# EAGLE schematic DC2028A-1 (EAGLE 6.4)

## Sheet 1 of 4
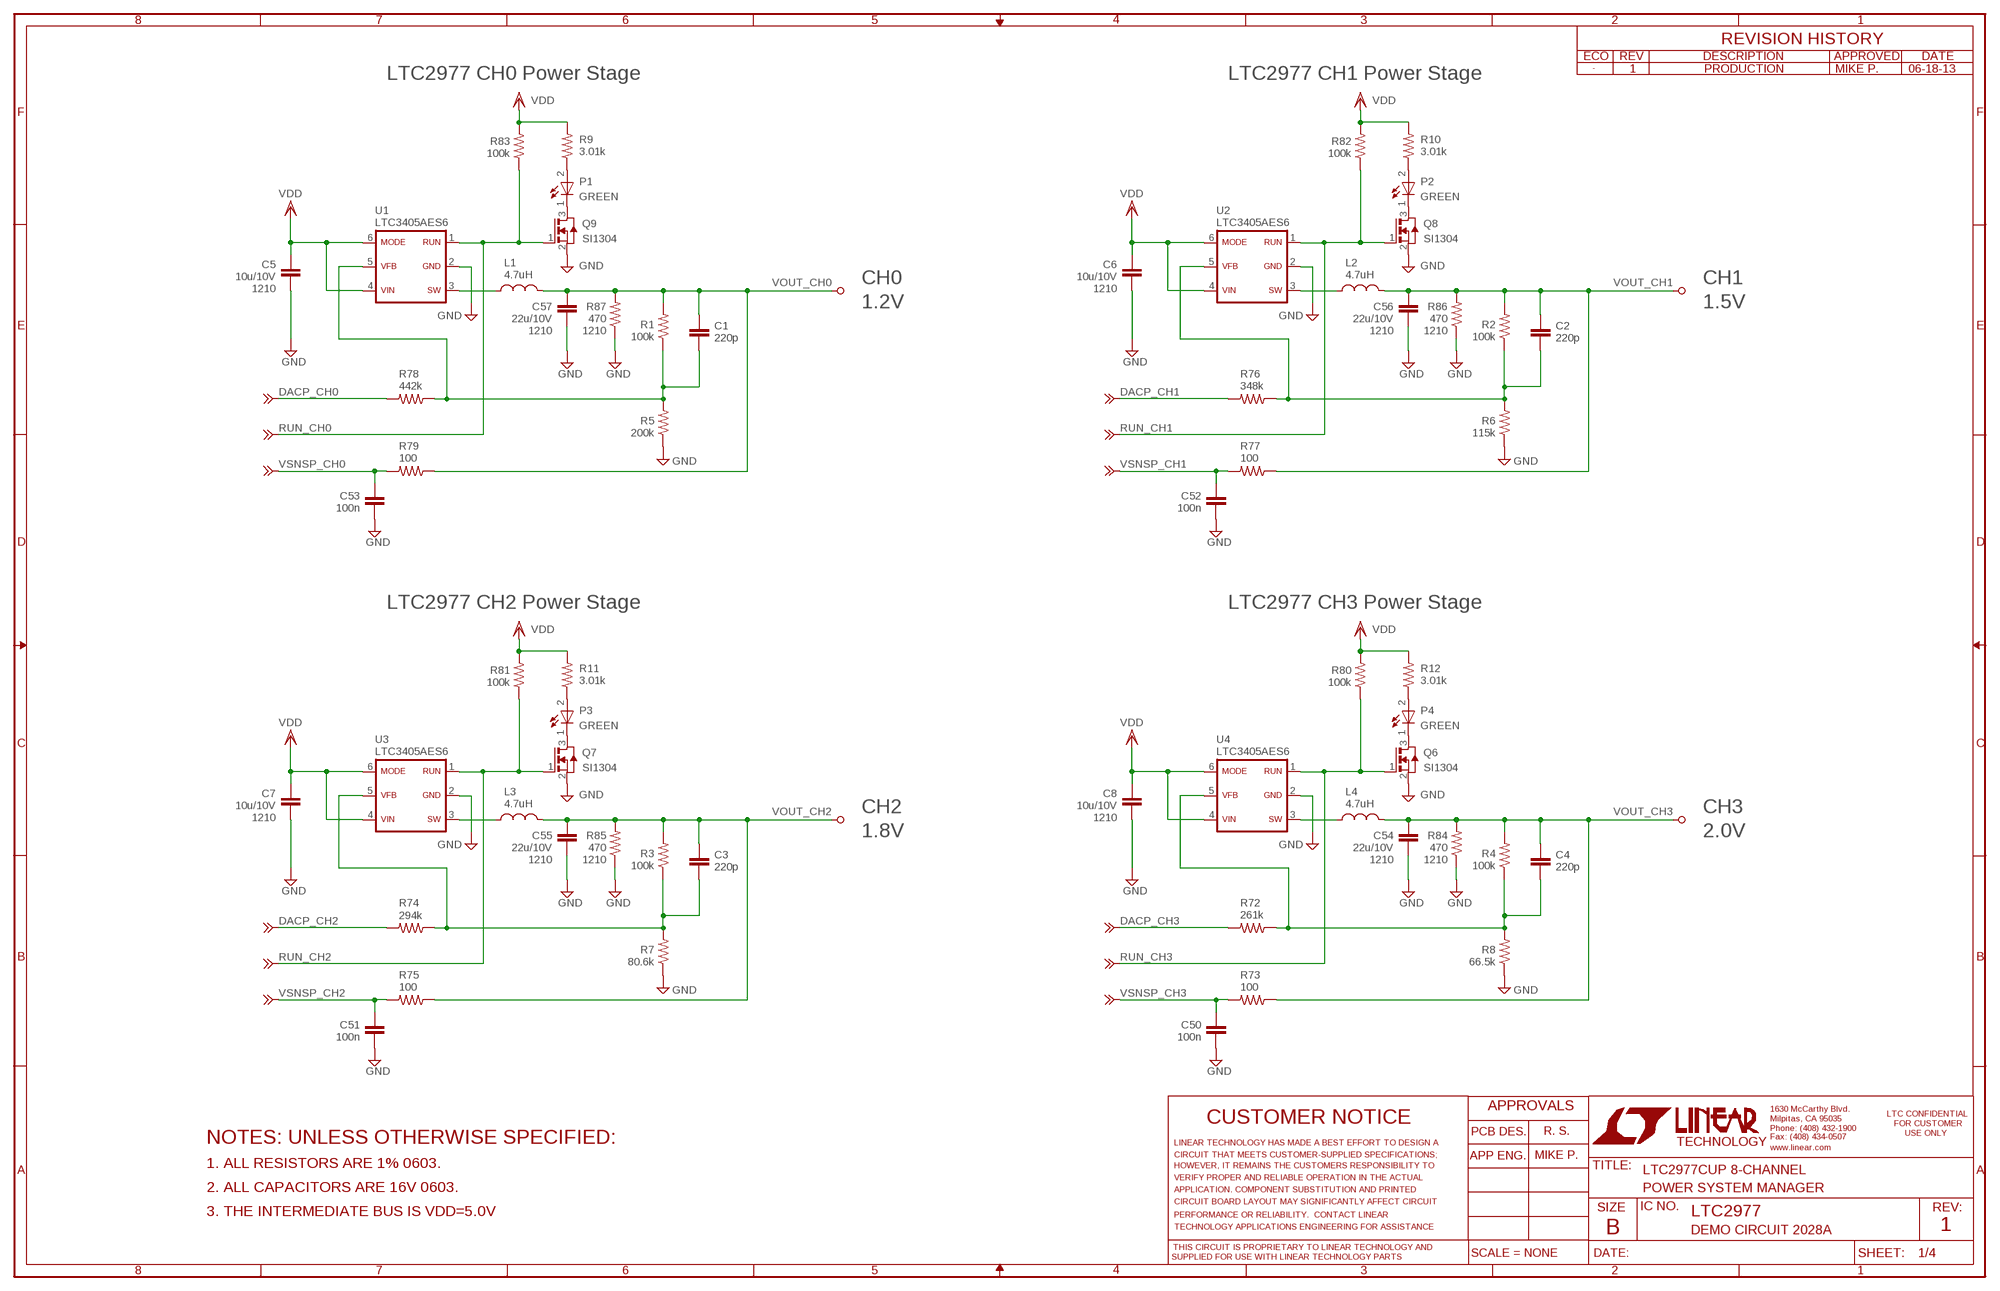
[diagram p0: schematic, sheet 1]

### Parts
C1  220p  CC0603_BOX  [C0603_BOX]
C2  220p  CC0603_BOX  [C0603_BOX]
C3  220p  CC0603_BOX  [C0603_BOX]
C4  220p  CC0603_BOX  [C0603_BOX]
C5  10u/10V  CC1210_BOX  [C1210_BOX]
C6  10u/10V  CC1210_BOX  [C1210_BOX]
C7  10u/10V  CC1210_BOX  [C1210_BOX]
C8  10u/10V  CC1210_BOX  [C1210_BOX]
C50  100n  CC0603_BOX  [C0603_BOX]
C51  100n  CC0603_BOX  [C0603_BOX]
C52  100n  CC0603_BOX  [C0603_BOX]
C53  100n  CC0603_BOX  [C0603_BOX]
C54  22u/10V  CC1210_BOX  [C1210_BOX]
C55  22u/10V  CC1210_BOX  [C1210_BOX]
C56  22u/10V  CC1210_BOX  [C1210_BOX]
C57  22u/10V  CC1210_BOX  [C1210_BOX]
L1  4.7uH  LL1210  [L1210]
L2  4.7uH  LL1210  [L1210]
L3  4.7uH  LL1210  [L1210]
L4  4.7uH  LL1210  [L1210]
P1  GREEN  LED-0603  [CHIPLED_0603]
P2  GREEN  LED-0603  [CHIPLED_0603]
P3  GREEN  LED-0603  [CHIPLED_0603]
P4  GREEN  LED-0603  [CHIPLED_0603]
Q6  SI1304  [SC70-3]
Q7  SI1304  [SC70-3]
Q8  SI1304  [SC70-3]
Q9  SI1304  [SC70-3]
R1  100k  RR0603_BOX  [R0603_BOX]
R2  100k  RR0603_BOX  [R0603_BOX]
R3  100k  RR0603_BOX  [R0603_BOX]
R4  100k  RR0603_BOX  [R0603_BOX]
R5  200k  RR0603_BOX  [R0603_BOX]
R6  115k  RR0603_BOX  [R0603_BOX]
R7  80.6k  RR0603_BOX  [R0603_BOX]
R8  66.5k  RR0603_BOX  [R0603_BOX]
R9  3.01k  RR0603_BOX  [R0603_BOX]
R10  3.01k  RR0603_BOX  [R0603_BOX]
R11  3.01k  RR0603_BOX  [R0603_BOX]
R12  3.01k  RR0603_BOX  [R0603_BOX]
R72  261k  RR0603_BOX  [R0603_BOX]
R73  100  RR0603_BOX  [R0603_BOX]
R74  294k  RR0603_BOX  [R0603_BOX]
R75  100  RR0603_BOX  [R0603_BOX]
R76  348k  RR0603_BOX  [R0603_BOX]
R77  100  RR0603_BOX  [R0603_BOX]
R78  442k  RR0603_BOX  [R0603_BOX]
R79  100  RR0603_BOX  [R0603_BOX]
R80  100k  RR0603_BOX  [R0603_BOX]
R81  100k  RR0603_BOX  [R0603_BOX]
R82  100k  RR0603_BOX  [R0603_BOX]
R83  100k  RR0603_BOX  [R0603_BOX]
R84  470  RR1210_BOX  [R1210_BOX]
R85  470  RR1210_BOX  [R1210_BOX]
R86  470  RR1210_BOX  [R1210_BOX]
R87  470  RR1210_BOX  [R1210_BOX]
TP3  TESTPOINT_BIG  [TP1]
TP4  TESTPOINT_BIG  [TP1]
TP5  TESTPOINT_BIG  [TP1]
TP6  TESTPOINT_BIG  [TP1]
U1  LTC3405AES6  LTC3405ES6  [SOT-23-6]
U2  LTC3405AES6  LTC3405ES6  [SOT-23-6]
U3  LTC3405AES6  LTC3405ES6  [SOT-23-6]
U4  LTC3405AES6  LTC3405ES6  [SOT-23-6]
VSNSN1  TESPOINT_SMD  TESPOINT_SMDVIA  [VIA]
VSNSN2  TESPOINT_SMD  TESPOINT_SMDVIA  [VIA]
VSNSN3  TESPOINT_SMD  TESPOINT_SMDVIA  [VIA]
VSNSN4  TESPOINT_SMD  TESPOINT_SMDVIA  [VIA]
VSNSN17  TESPOINT_SMD  TESPOINT_SMDVIA  [VIA]
VSNSN18  TESPOINT_SMD  TESPOINT_SMDVIA  [VIA]
VSNSN19  TESPOINT_SMD  TESPOINT_SMDVIA  [VIA]
VSNSN20  TESPOINT_SMD  TESPOINT_SMDVIA  [VIA]
VSNSN21  TESPOINT_SMD  TESPOINT_SMDVIA  [VIA]
VSNSN22  TESPOINT_SMD  TESPOINT_SMDVIA  [VIA]
VSNSN23  TESPOINT_SMD  TESPOINT_SMDVIA  [VIA]
VSNSN24  TESPOINT_SMD  TESPOINT_SMDVIA  [VIA]

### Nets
DACP_CH0: R78.2 VSNSN23.1 ; also sheet 3
DACP_CH1: R76.2 VSNSN21.1 ; also sheet 3
DACP_CH2: R74.2 VSNSN19.1 ; also sheet 3
DACP_CH3: R72.2 VSNSN17.1 ; also sheet 3
GND: C5.2 C6.2 C7.2 C8.2 C50.1 C51.1 C52.1 C53.1 C54.2 C55.2 C56.2 C57.2 Q6.2(S) Q7.2(S) Q8.2(S) Q9.2(S) R5.1 R6.1 R7.1 R8.1 R84.1 R85.1 R86.1 R87.1 U1.2 U2.2 U3.2 U4.2 ; also sheet 2,3,4
N$6: P1.P(A) R9.1
N$7: P1.N(C) Q9.3(D)
N$8: P2.P(A) R10.1
N$9: P2.N(C) Q8.3(D)
N$10: P3.P(A) R11.1
N$11: P3.N(C) Q7.3(D)
N$12: P4.P(A) R12.1
N$13: P4.N(C) Q6.3(D)
RUN_CH0: Q9.1(G) R83.1 U1.1 VSNSN1.1 ; also sheet 3
RUN_CH1: Q8.1(G) R82.1 U2.1 VSNSN2.1 ; also sheet 3
RUN_CH2: Q7.1(G) R81.1 U3.1 VSNSN3.1 ; also sheet 3
RUN_CH3: Q6.1(G) R80.1 U4.1 VSNSN4.1 ; also sheet 3
SW1: L1.1 U1.3
SW2: L2.1 U2.3
SW3: L3.1 U3.3
SW4: L4.1 U4.3
VDD: C5.1 C6.1 C7.1 C8.1 R9.2 R10.2 R11.2 R12.2 R80.2 R81.2 R82.2 R83.2 U1.4 U1.6 U2.4 U2.6 U3.4 U3.6 U4.4 U4.6 ; also sheet 2,3,4
VFB1: C1.2 R1.1 R5.2 R78.1 U1.5
VFB2: C2.2 R2.1 R6.2 R76.1 U2.5
VFB3: C3.2 R3.1 R7.2 R74.1 U3.5
VFB12: C4.2 R4.1 R8.2 R72.1 U4.5
VOUT_CH0: C1.1 C57.1 L1.2 R1.2 R79.1 R87.2 TP3.TP
VOUT_CH1: C2.1 C56.1 L2.2 R2.2 R77.1 R86.2 TP4.TP
VOUT_CH2: C3.1 C55.1 L3.2 R3.2 R75.1 R85.2 TP5.TP
VOUT_CH3: C4.1 C54.1 L4.2 R4.2 R73.1 R84.2 TP6.TP
VSNSP_CH0: C53.2 R79.2 VSNSN24.1 ; also sheet 3
VSNSP_CH1: C52.2 R77.2 VSNSN22.1 ; also sheet 3
VSNSP_CH2: C51.2 R75.2 VSNSN20.1 ; also sheet 3
VSNSP_CH3: C50.2 R73.2 VSNSN18.1 ; also sheet 3

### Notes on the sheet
- 1 | PRODUCTION | MIKE P. | 06-18-13
- LTC2977 CH0 Power Stage | LTC2977 CH1 Power Stage
- 1210 | CH0 | 1210 | CH1
- 1.2V | 1.5V
- 1210 | 1210 | 1210 | 1210
- LTC2977 CH2 Power Stage | LTC2977 CH3 Power Stage
- 1210 | CH2 | 1210 | CH3
- 1.8V | 2.0V
- 1210 | 1210 | 1210 | 1210
- R. S.
- NOTES: UNLESS OTHERWISE SPECIFIED:
- MIKE P.
- 1. ALL RESISTORS ARE 1% 0603.
- LTC2977CUP 8-CHANNEL
- 2. ALL CAPACITORS ARE 16V 0603. | POWER SYSTEM MANAGER
- 3. THE INTERMEDIATE BUS IS VDD=5.0V | LTC2977
- DEMO CIRCUIT 2028A | 1

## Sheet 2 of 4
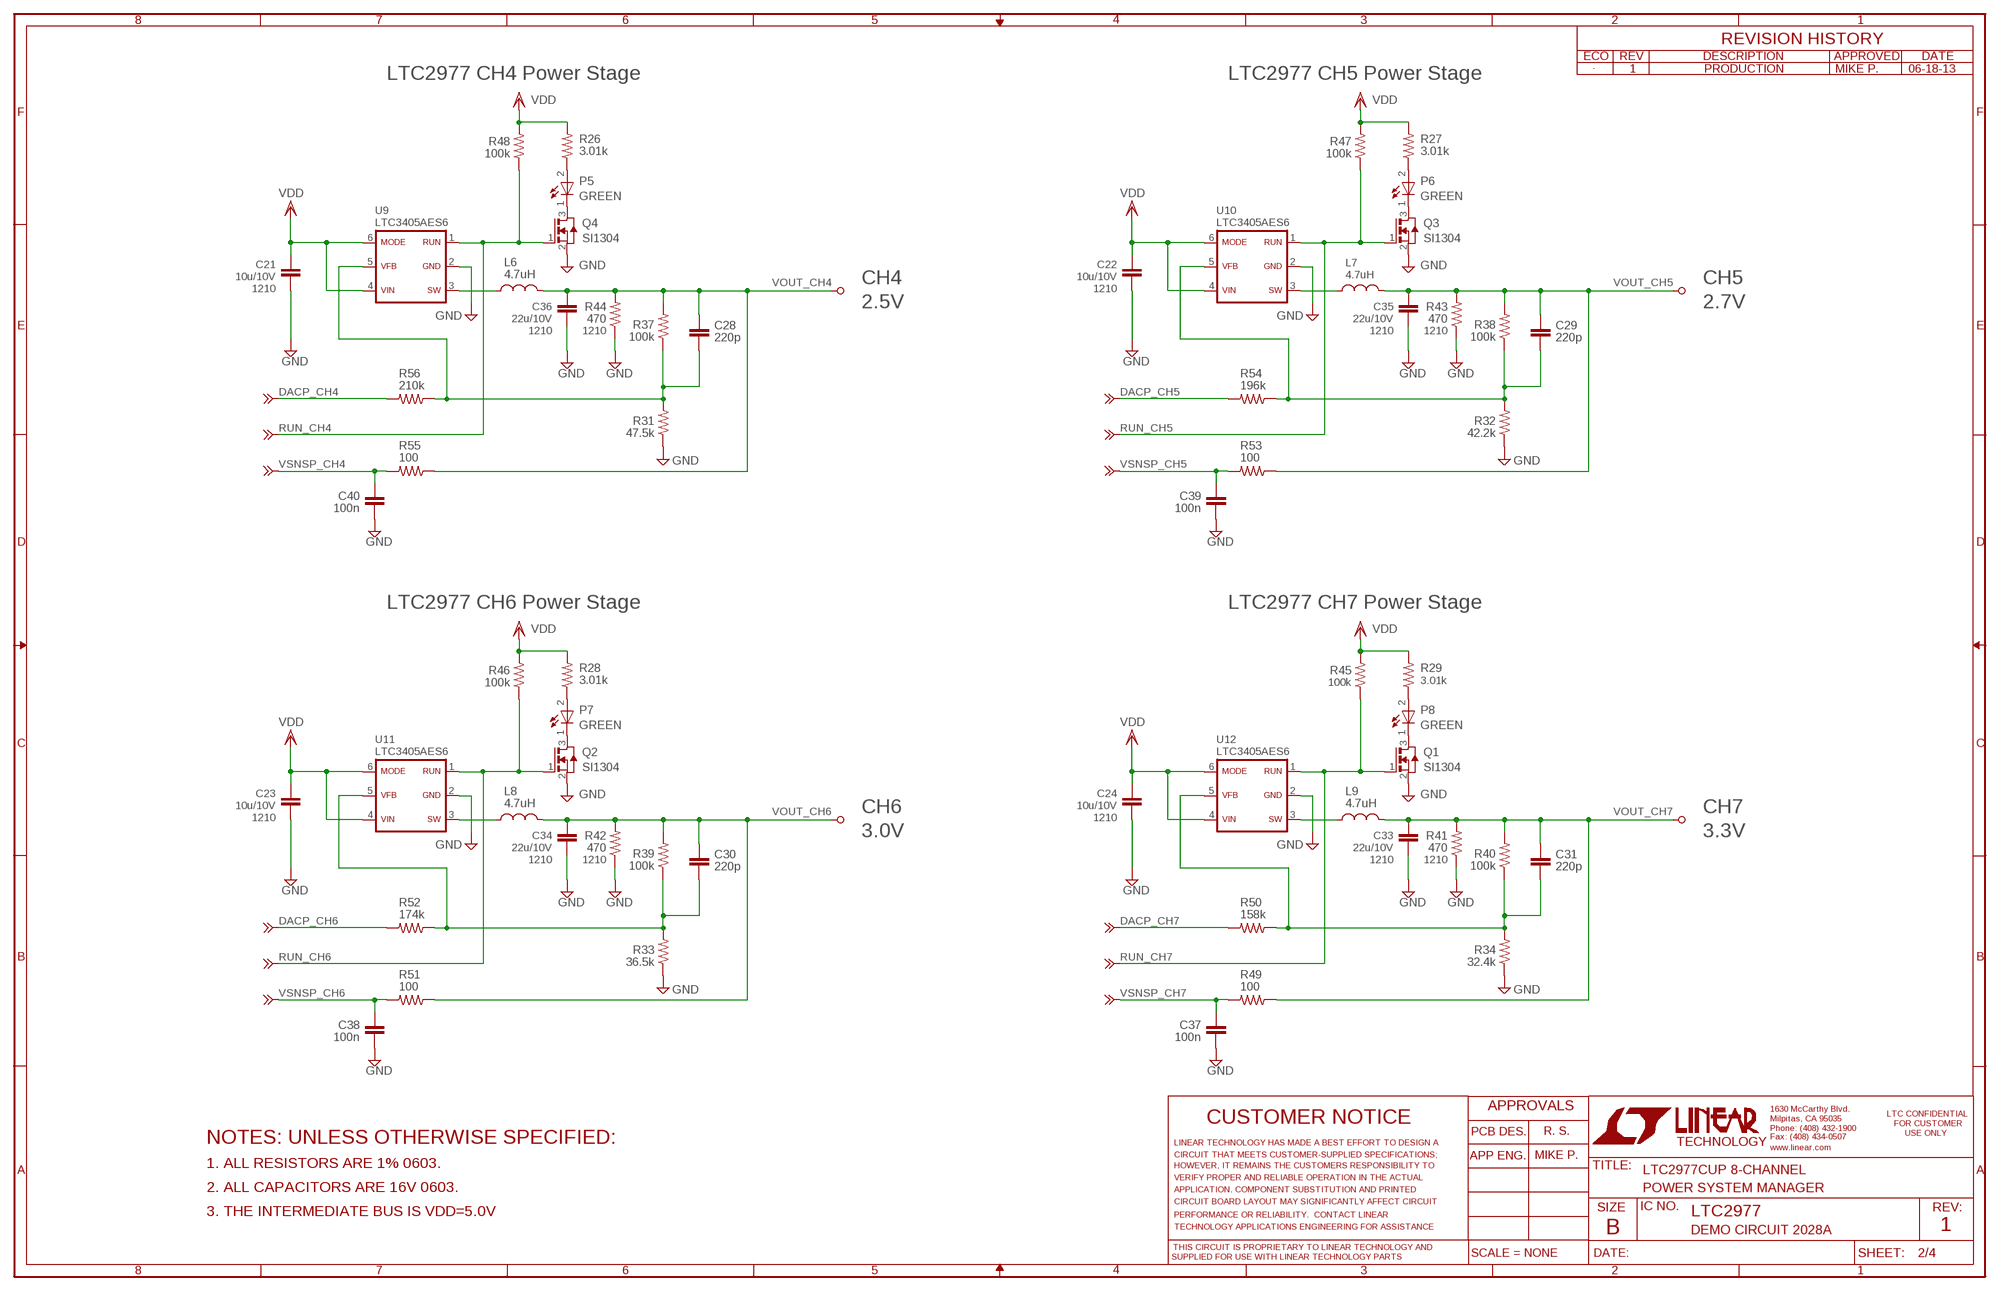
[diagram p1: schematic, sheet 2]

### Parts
C21  10u/10V  CC1210_BOX  [C1210_BOX]
C22  10u/10V  CC1210_BOX  [C1210_BOX]
C23  10u/10V  CC1210_BOX  [C1210_BOX]
C24  10u/10V  CC1210_BOX  [C1210_BOX]
C28  220p  CC0603_BOX  [C0603_BOX]
C29  220p  CC0603_BOX  [C0603_BOX]
C30  220p  CC0603_BOX  [C0603_BOX]
C31  220p  CC0603_BOX  [C0603_BOX]
C33  22u/10V  CC1210_BOX  [C1210_BOX]
C34  22u/10V  CC1210_BOX  [C1210_BOX]
C35  22u/10V  CC1210_BOX  [C1210_BOX]
C36  22u/10V  CC1210_BOX  [C1210_BOX]
C37  100n  CC0603_BOX  [C0603_BOX]
C38  100n  CC0603_BOX  [C0603_BOX]
C39  100n  CC0603_BOX  [C0603_BOX]
C40  100n  CC0603_BOX  [C0603_BOX]
L6  4.7uH  LL1210  [L1210]
L7  4.7uH  LL1210  [L1210]
L8  4.7uH  LL1210  [L1210]
L9  4.7uH  LL1210  [L1210]
P5  GREEN  LED-0603  [CHIPLED_0603]
P6  GREEN  LED-0603  [CHIPLED_0603]
P7  GREEN  LED-0603  [CHIPLED_0603]
P8  GREEN  LED-0603  [CHIPLED_0603]
Q1  SI1304  [SC70-3]
Q2  SI1304  [SC70-3]
Q3  SI1304  [SC70-3]
Q4  SI1304  [SC70-3]
R26  3.01k  RR0603_BOX  [R0603_BOX]
R27  3.01k  RR0603_BOX  [R0603_BOX]
R28  3.01k  RR0603_BOX  [R0603_BOX]
R29  3.01k  RR0603_BOX  [R0603_BOX]
R31  47.5k  RR0603_BOX  [R0603_BOX]
R32  42.2k  RR0603_BOX  [R0603_BOX]
R33  36.5k  RR0603_BOX  [R0603_BOX]
R34  32.4k  RR0603_BOX  [R0603_BOX]
R37  100k  RR0603_BOX  [R0603_BOX]
R38  100k  RR0603_BOX  [R0603_BOX]
R39  100k  RR0603_BOX  [R0603_BOX]
R40  100k  RR0603_BOX  [R0603_BOX]
R41  470  RR1210_BOX  [R1210_BOX]
R42  470  RR1210_BOX  [R1210_BOX]
R43  470  RR1210_BOX  [R1210_BOX]
R44  470  RR1210_BOX  [R1210_BOX]
R45  100k  RR0603_BOX  [R0603_BOX]
R46  100k  RR0603_BOX  [R0603_BOX]
R47  100k  RR0603_BOX  [R0603_BOX]
R48  100k  RR0603_BOX  [R0603_BOX]
R49  100  RR0603_BOX  [R0603_BOX]
R50  158k  RR0603_BOX  [R0603_BOX]
R51  100  RR0603_BOX  [R0603_BOX]
R52  174k  RR0603_BOX  [R0603_BOX]
R53  100  RR0603_BOX  [R0603_BOX]
R54  196k  RR0603_BOX  [R0603_BOX]
R55  100  RR0603_BOX  [R0603_BOX]
R56  210k  RR0603_BOX  [R0603_BOX]
TP17  TESTPOINT_BIG  [TP1]
TP18  TESTPOINT_BIG  [TP1]
TP19  TESTPOINT_BIG  [TP1]
TP20  TESTPOINT_BIG  [TP1]
U9  LTC3405AES6  LTC3405ES6  [SOT-23-6]
U10  LTC3405AES6  LTC3405ES6  [SOT-23-6]
U11  LTC3405AES6  LTC3405ES6  [SOT-23-6]
U12  LTC3405AES6  LTC3405ES6  [SOT-23-6]
VSNSN5  TESPOINT_SMD  TESPOINT_SMDVIA  [VIA]
VSNSN6  TESPOINT_SMD  TESPOINT_SMDVIA  [VIA]
VSNSN7  TESPOINT_SMD  TESPOINT_SMDVIA  [VIA]
VSNSN8  TESPOINT_SMD  TESPOINT_SMDVIA  [VIA]
VSNSN9  TESPOINT_SMD  TESPOINT_SMDVIA  [VIA]
VSNSN10  TESPOINT_SMD  TESPOINT_SMDVIA  [VIA]
VSNSN11  TESPOINT_SMD  TESPOINT_SMDVIA  [VIA]
VSNSN12  TESPOINT_SMD  TESPOINT_SMDVIA  [VIA]
VSNSN13  TESPOINT_SMD  TESPOINT_SMDVIA  [VIA]
VSNSN14  TESPOINT_SMD  TESPOINT_SMDVIA  [VIA]
VSNSN15  TESPOINT_SMD  TESPOINT_SMDVIA  [VIA]
VSNSN16  TESPOINT_SMD  TESPOINT_SMDVIA  [VIA]

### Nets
DACP_CH4: R56.2 VSNSN16.1 ; also sheet 3
DACP_CH5: R54.2 VSNSN14.1 ; also sheet 3
DACP_CH6: R52.2 VSNSN12.1 ; also sheet 3
DACP_CH7: R50.2 VSNSN10.1 ; also sheet 3
GND: C21.2 C22.2 C23.2 C24.2 C33.2 C34.2 C35.2 C36.2 C37.1 C38.1 C39.1 C40.1 Q1.2(S) Q2.2(S) Q3.2(S) Q4.2(S) R31.1 R32.1 R33.1 R34.1 R41.1 R42.1 R43.1 R44.1 U9.2 U10.2 U11.2 U12.2 ; also sheet 1,3,4
N$29: P5.P(A) R26.1
N$30: P5.N(C) Q4.3(D)
N$31: P6.P(A) R27.1
N$32: P6.N(C) Q3.3(D)
N$33: P7.P(A) R28.1
N$34: P7.N(C) Q2.3(D)
N$35: P8.P(A) R29.1
N$36: P8.N(C) Q1.3(D)
RUN_CH4: Q4.1(G) R48.1 U9.1 VSNSN5.1 ; also sheet 3
RUN_CH5: Q3.1(G) R47.1 U10.1 VSNSN6.1 ; also sheet 3
RUN_CH6: Q2.1(G) R46.1 U11.1 VSNSN7.1 ; also sheet 3
RUN_CH7: Q1.1(G) R45.1 U12.1 VSNSN8.1 ; also sheet 3
SW11: L6.1 U9.3
SW12: L7.1 U10.3
SW13: L8.1 U11.3
SW14: L9.1 U12.3
VDD: C21.1 C22.1 C23.1 C24.1 R26.2 R27.2 R28.2 R29.2 R45.2 R46.2 R47.2 R48.2 U9.4 U9.6 U10.4 U10.6 U11.4 U11.6 U12.4 U12.6 ; also sheet 1,3,4
VFB4: C28.2 R31.2 R37.1 R56.1 U9.5
VFB5: C29.2 R32.2 R38.1 R54.1 U10.5
VFB6: C30.2 R33.2 R39.1 R52.1 U11.5
VFB7: C31.2 R34.2 R40.1 R50.1 U12.5
VOUT_CH4: C28.1 C36.1 L6.2 R37.2 R44.2 R55.1 TP17.TP
VOUT_CH5: C29.1 C35.1 L7.2 R38.2 R43.2 R53.1 TP18.TP
VOUT_CH6: C30.1 C34.1 L8.2 R39.2 R42.2 R51.1 TP19.TP
VOUT_CH7: C31.1 C33.1 L9.2 R40.2 R41.2 R49.1 TP20.TP ; also sheet 3
VSNSP_CH4: C40.2 R55.2 VSNSN15.1 ; also sheet 3
VSNSP_CH5: C39.2 R53.2 VSNSN13.1 ; also sheet 3
VSNSP_CH6: C38.2 R51.2 VSNSN11.1 ; also sheet 3
VSNSP_CH7: C37.2 R49.2 VSNSN9.1 ; also sheet 3

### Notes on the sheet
- 1 | PRODUCTION | MIKE P. | 06-18-13
- LTC2977 CH4 Power Stage | LTC2977 CH5 Power Stage
- 1210 | CH4 | 1210 | CH5
- 2.5V | 2.7V
- 1210 | 1210 | 1210 | 1210
- LTC2977 CH6 Power Stage | LTC2977 CH7 Power Stage
- 1210 | CH6 | 1210 | CH7
- 3.0V | 3.3V
- 1210 | 1210 | 1210 | 1210
- R. S.
- NOTES: UNLESS OTHERWISE SPECIFIED:
- MIKE P.
- 1. ALL RESISTORS ARE 1% 0603.
- LTC2977CUP 8-CHANNEL
- 2. ALL CAPACITORS ARE 16V 0603. | POWER SYSTEM MANAGER
- 3. THE INTERMEDIATE BUS IS VDD=5.0V | LTC2977
- DEMO CIRCUIT 2028A | 1

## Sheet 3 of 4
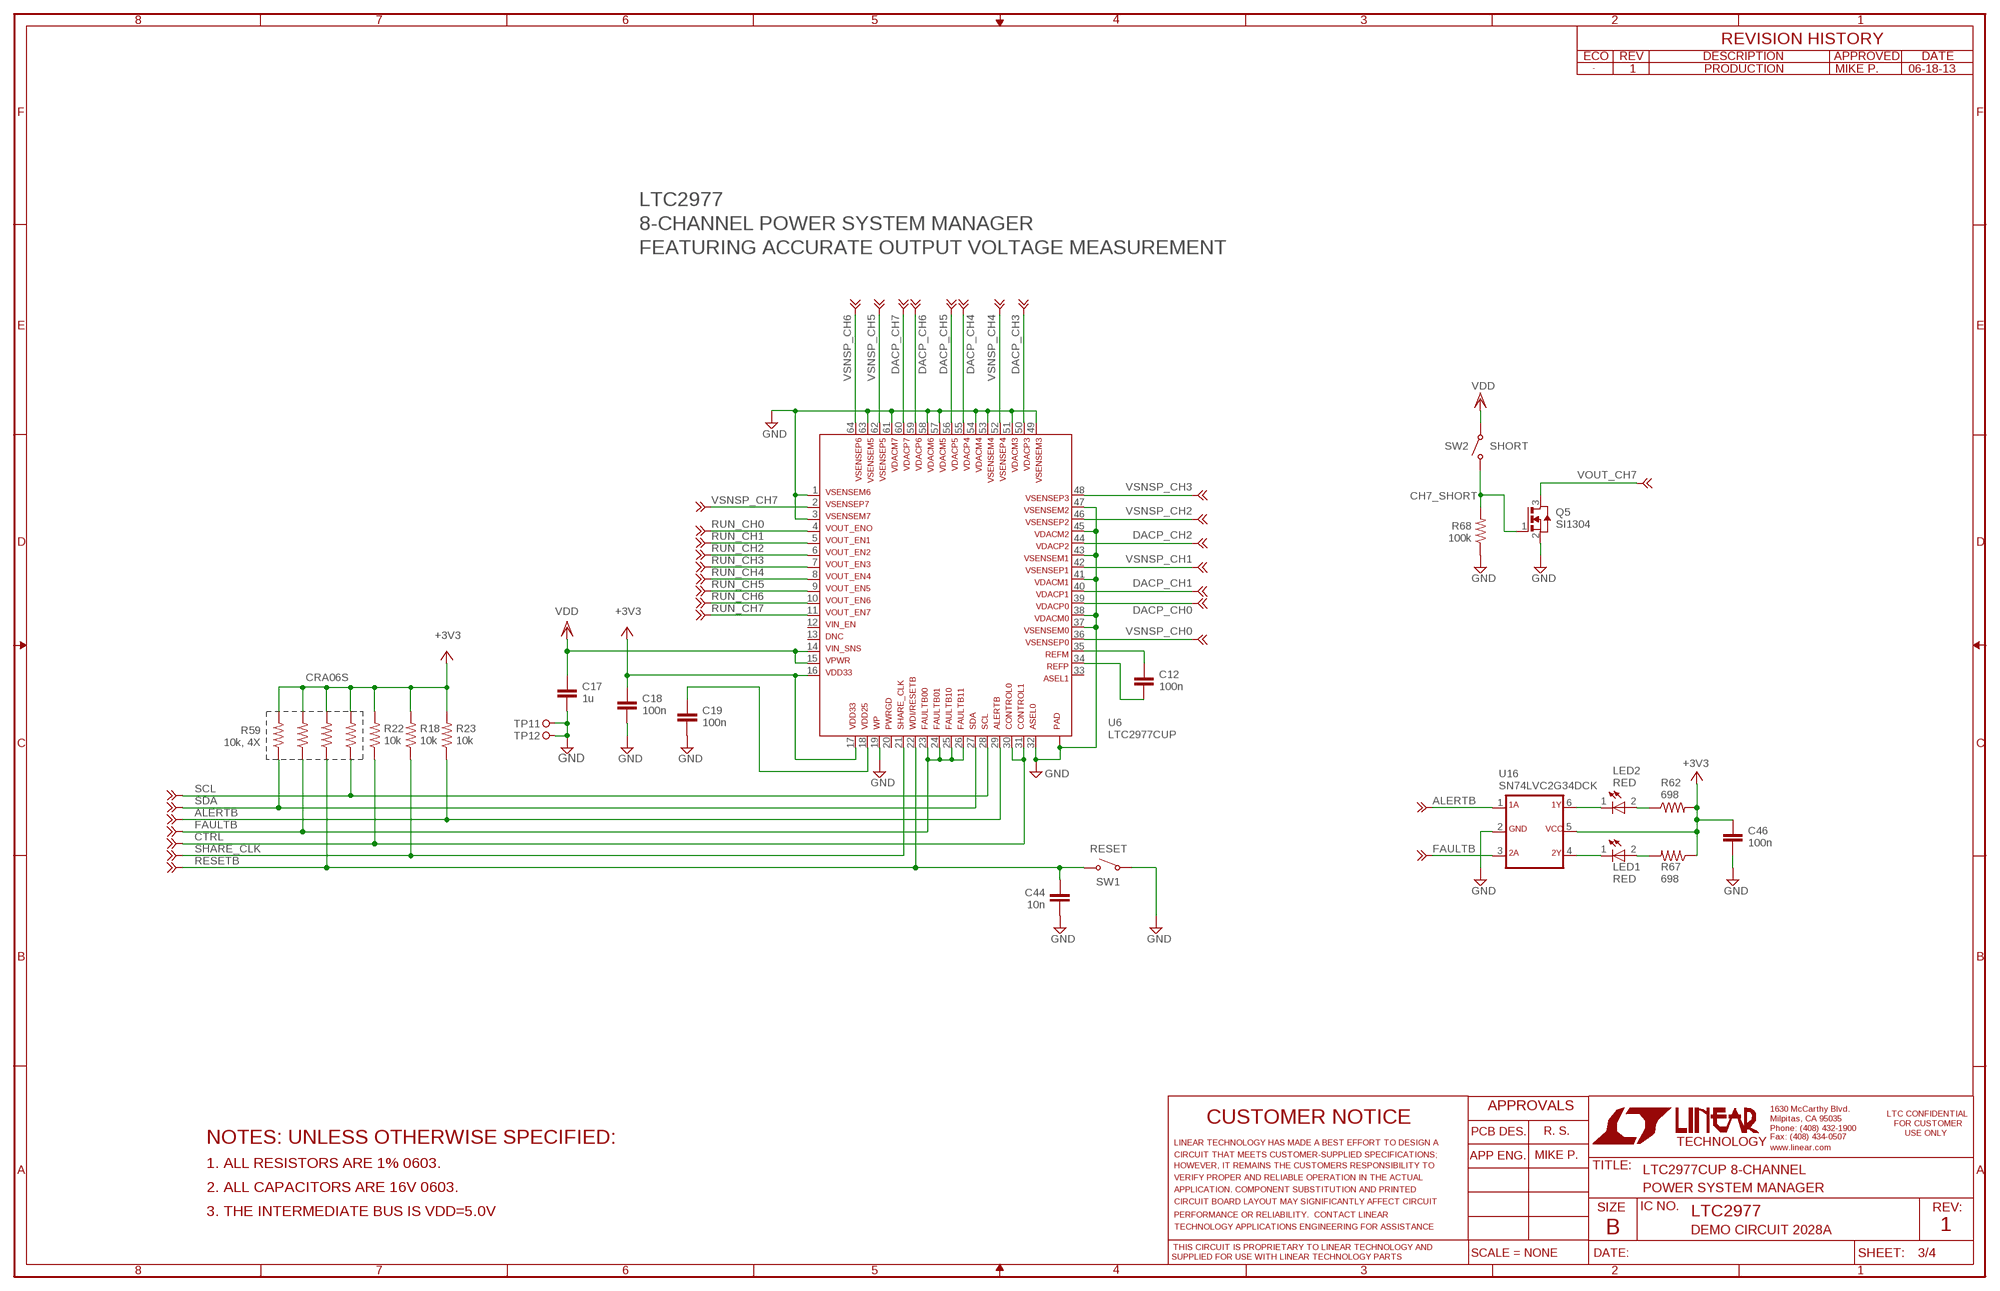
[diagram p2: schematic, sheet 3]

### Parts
C12  100n  CC0603_BOX  [C0603_BOX]
C17  1u  CC0603_BOX  [C0603_BOX]
C18  100n  CC0603_BOX  [C0603_BOX]
C19  100n  CC0603_BOX  [C0603_BOX]
C44  10n  CC0603_BOX  [C0603_BOX]
C46  100n  CC0603_BOX  [C0603_BOX]
LED1  RED  LED-0603  [CHIPLED_0603]
LED2  RED  LED-0603  [CHIPLED_0603]
Q5  SI1304  [SC70-3]
R18  10k  RR0603_BOX  [R0603_BOX]
R22  10k  RR0603_BOX  [R0603_BOX]
R23  10k  RR0603_BOX  [R0603_BOX]
R59  10k, 4X  R_ARRAY_4X_CRA06S  [R_VISHAY_CRA06S]
R62  698  RR0603_BOX  [R0603_BOX]
R67  698  RR0603_BOX  [R0603_BOX]
R68  100k  RR0603_BOX  [R0603_BOX]
SW1  PTS635SL25SMTR LFS  SWITCH_PTS635  [SWITCH_PTS635]
SW2  PTS635SK25SMTR LFS  SWITCH_PTS635  [SWITCH_PTS635]
TP11  TESTPOINT_BIG  [TP1]
TP12  TESTPOINT_BIG  [TP1]
U6  LTC2977CUP  LTC2978CUP  [QFN64_9X9]
U16  SN74LVC2G34DCK  [SC70-6]

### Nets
+3V3: C18.2 C46.1 R18.2 R22.2 R23.2 R59.R1_2 R59.R2_2 R59.R3_2 R59.R4_2 R62.2 R67.1 U6.16 U6.17 U16.5 ; also sheet 4
ALERTB: R23.1 U6.29 U16.1 ; also sheet 4
CH7_SHORT: Q5.1(G) R68.2 SW2.SW1 ; also sheet 4
CTRL: R22.1 U6.30 U6.31 ; also sheet 4
DACP_CH0: U6.39 ; also sheet 1
DACP_CH1: U6.40 ; also sheet 1
DACP_CH2: U6.44 ; also sheet 1
DACP_CH3: U6.50 ; also sheet 1
DACP_CH4: U6.55 ; also sheet 2
DACP_CH5: U6.56 ; also sheet 2
DACP_CH6: U6.59 ; also sheet 2
DACP_CH7: U6.60 ; also sheet 2
FAULTB: R59.R2_1 U6.23 U6.24 U6.25 U6.26 U16.3 ; also sheet 4
GND: C17.1 C18.1 C19.1 C44.2 C46.2 Q5.2(S) R68.1 SW1.SW2 TP11.TP TP12.TP U6.1 U6.3 U6.19 U6.32 U6.37 U6.38 U6.41 U6.43 U6.45 U6.47 U6.49 U6.51 U6.53 U6.54 U6.57 U6.58 U6.61 U6.63 U6.PAD1 U6.PAD2 U6.PAD3 U6.PAD4 U16.2 ; also sheet 1,2,4
N$3: LED1.P(A) R67.2
N$53: C12.1 U6.35
N$54: C12.2 U6.34
N$56: C19.2 U6.18
N$57: LED2.P(A) R62.1
N$58: LED1.N(C) U16.4
N$60: LED2.N(C) U16.6
RESETB: C44.1 R59.R3_1 SW1.SW1 U6.22 ; also sheet 4
RUN_CH0: U6.4 ; also sheet 1
RUN_CH1: U6.5 ; also sheet 1
RUN_CH2: U6.6 ; also sheet 1
RUN_CH3: U6.7 ; also sheet 1
RUN_CH4: U6.8 ; also sheet 2
RUN_CH5: U6.9 ; also sheet 2
RUN_CH6: U6.10 ; also sheet 2
RUN_CH7: U6.11 ; also sheet 2
SCL: R59.R4_1 U6.28 ; also sheet 4
SDA: R59.R1_1 U6.27 ; also sheet 4
SHARE_CLK: R18.1 U6.21 ; also sheet 4
VDD: C17.2 SW2.SW2 U6.14 U6.15 ; also sheet 1,2,4
VOUT_CH7: Q5.3(D) ; also sheet 2
VSNSP_CH0: U6.36 ; also sheet 1
VSNSP_CH1: U6.42 ; also sheet 1
VSNSP_CH2: U6.46 ; also sheet 1
VSNSP_CH3: U6.48 ; also sheet 1
VSNSP_CH4: U6.52 ; also sheet 2
VSNSP_CH5: U6.62 ; also sheet 2
VSNSP_CH6: U6.64 ; also sheet 2
VSNSP_CH7: U6.2 ; also sheet 2
Unconnected: U6.12 U6.13 U6.20 U6.33

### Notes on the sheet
- 1 | PRODUCTION | MIKE P. | 06-18-13
- LTC2977
- 8-CHANNEL POWER SYSTEM MANAGER
- FEATURING ACCURATE OUTPUT VOLTAGE MEASUREMENT
- SHORT
- CRA06S
- RESET
- R. S.
- NOTES: UNLESS OTHERWISE SPECIFIED:
- MIKE P.
- 1. ALL RESISTORS ARE 1% 0603.
- LTC2977CUP 8-CHANNEL
- 2. ALL CAPACITORS ARE 16V 0603. | POWER SYSTEM MANAGER
- 3. THE INTERMEDIATE BUS IS VDD=5.0V | LTC2977
- DEMO CIRCUIT 2028A | 1

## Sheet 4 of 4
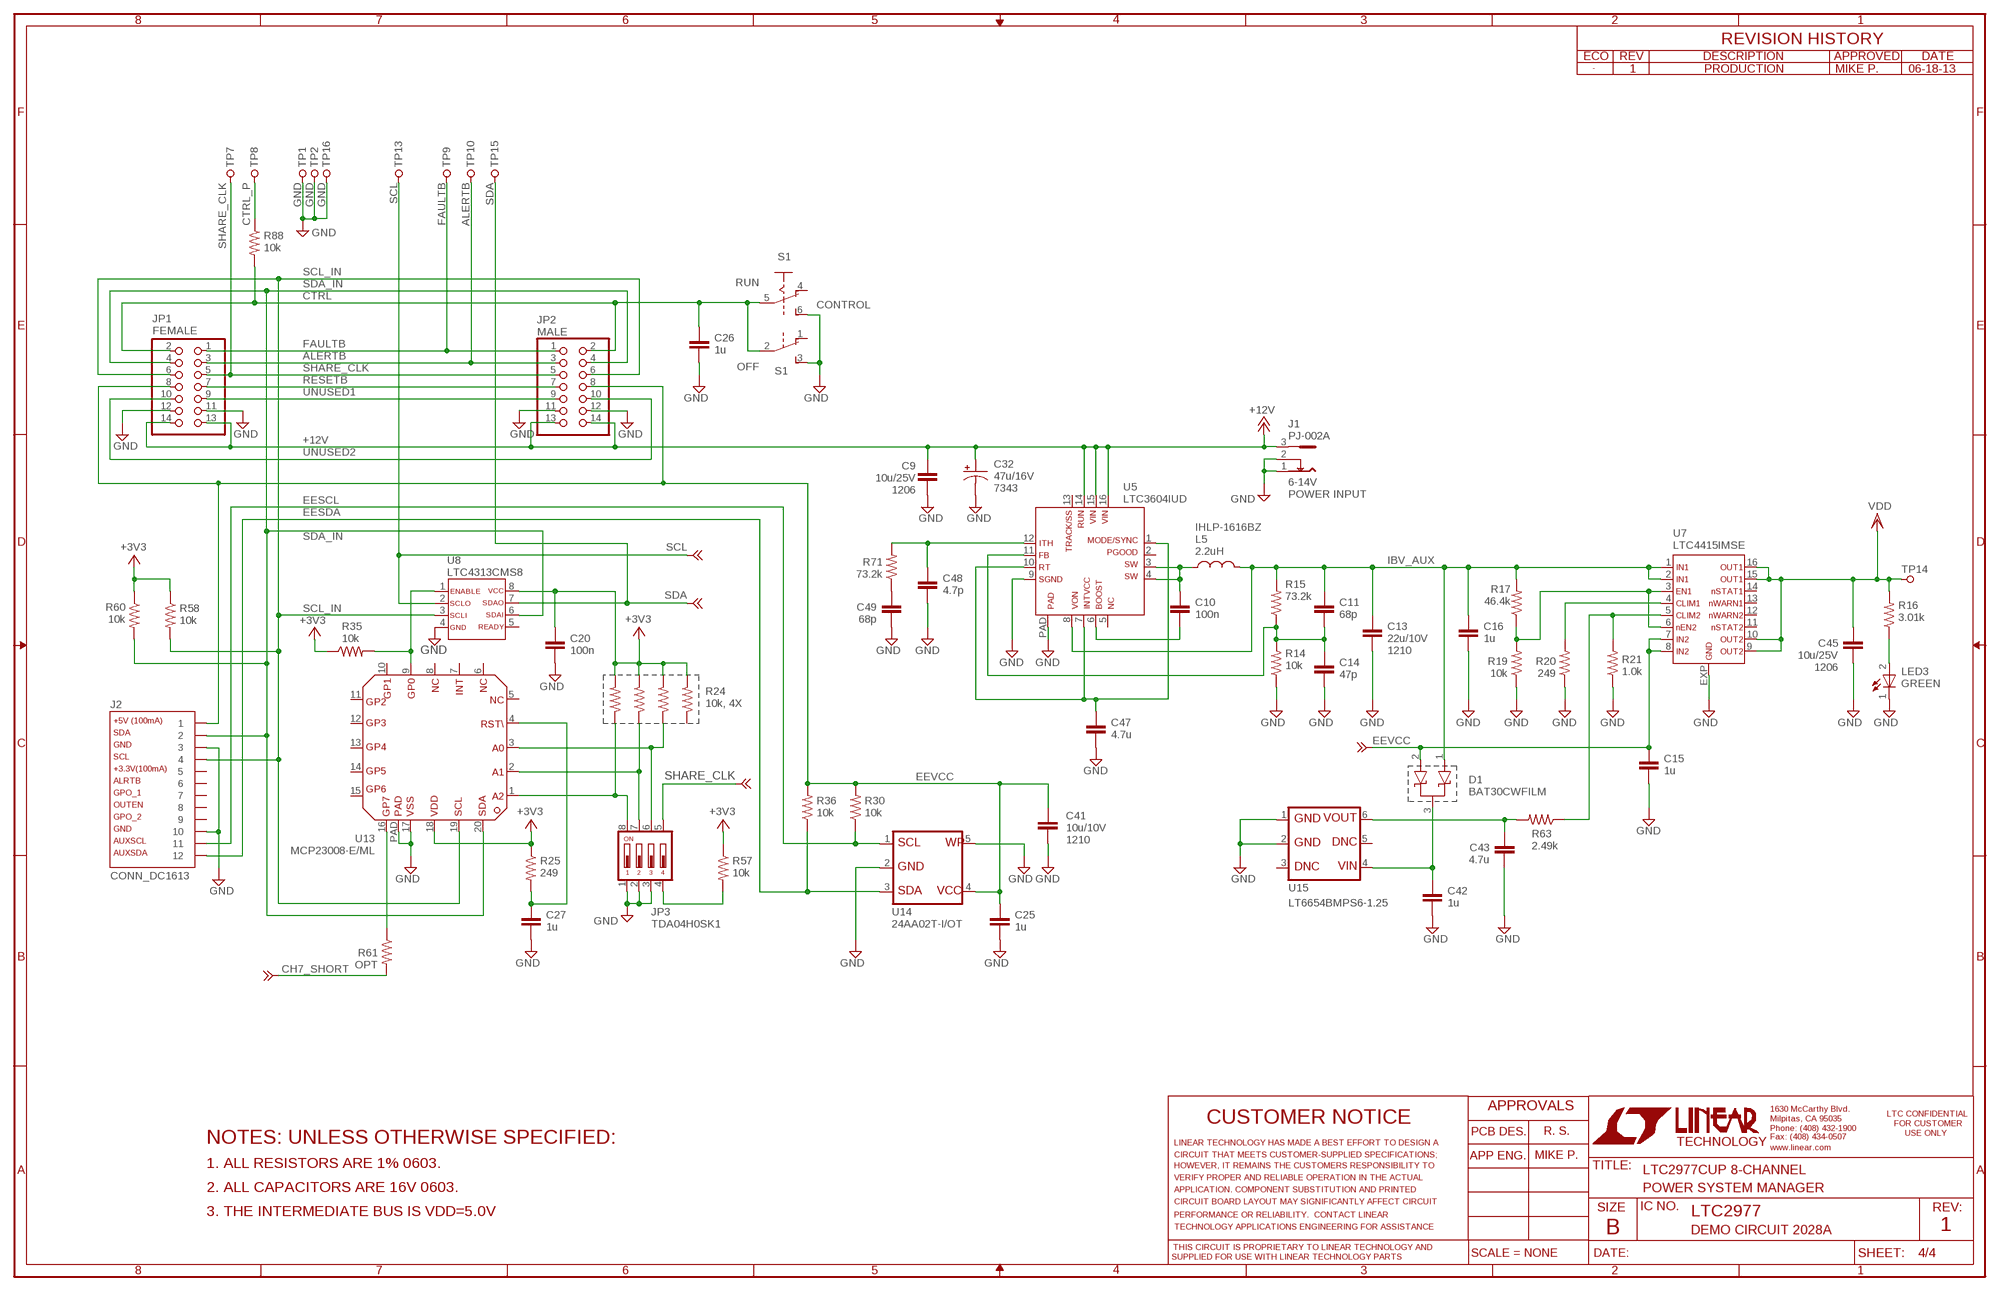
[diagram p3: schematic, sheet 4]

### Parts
C9  10u/25V  CC1206_BOX  [C1206_BOX]
C10  100n  CC0603_BOX  [C0603_BOX]
C11  68p  CC0603_BOX  [C0603_BOX]
C13  22u/10V  CC1210_BOX  [C1210_BOX]
C14  47p  CC0603_BOX  [C0603_BOX]
C15  1u  CC0603_BOX  [C0603_BOX]
C16  1u  CC0603_BOX  [C0603_BOX]
C20  100n  CC0603_BOX  [C0603_BOX]
C25  1u  CC0603_BOX  [C0603_BOX]
C26  1u  CC0603_BOX  [C0603_BOX]
C27  1u  CC0603_BOX  [C0603_BOX]
C32  47u/16V  CPOL  [C7343]
C41  10u/10V  CC1210_BOX  [C1210_BOX]
C42  1u  CC0603_BOX  [C0603_BOX]
C43  4.7u  CC0603_BOX  [C0603_BOX]
C45  10u/25V  CC1206_BOX  [C1206_BOX]
C47  4.7u  CC0603_BOX  [C0603_BOX]
C48  4.7p  CC0603_BOX  [C0603_BOX]
C49  68p  CC0603_BOX  [C0603_BOX]
D1  BAT30CWFILM  [SC70-3]
J1  PJ-002A  [PJ-002A]
J2  CONN_DC1613  [CONN_DC1613]
JP1  FEMALE  PINHD-2X07_2.00  [2X07M]
JP2  MALE  PINHD-2X07_2.00  [2X07M]
JP3  TDA04H0SK1  [SMT_DIP_4]
L5  2.2uH  LVISHAY-IHLP1616AB  [IHLP_1616AB]
LED3  GREEN  LED-0603  [CHIPLED_0603]
R14  10k  RR0603_BOX  [R0603_BOX]
R15  73.2k  RR0603_BOX  [R0603_BOX]
R16  3.01k  RR0603_BOX  [R0603_BOX]
R17  46.4k  RR0603_BOX  [R0603_BOX]
R19  10k  RR0603_BOX  [R0603_BOX]
R20  249  RR0603_BOX  [R0603_BOX]
R21  1.0k  RR0603_BOX  [R0603_BOX]
R24  10k, 4X  R_ARRAY_4X_CRA06S  [R_VISHAY_CRA06S]
R25  249  RR0603_BOX  [R0603_BOX]
R30  10k  RR0603_BOX  [R0603_BOX]
R35  10k  RR0603_BOX  [R0603_BOX]
R36  10k  RR0603_BOX  [R0603_BOX]
R57  10k  RR0603_BOX  [R0603_BOX]
R58  10k  RR0603_BOX  [R0603_BOX]
R60  10k  RR0603_BOX  [R0603_BOX]
R61  OPT  RR0603_BOX  [R0603_BOX]
R63  2.49k  RR0603_BOX  [R0603_BOX]
R71  73.2k  RR0603_BOX  [R0603_BOX]
R88  10k  RR0603_BOX  [R0603_BOX]
S1  CONTROL  JS202011CQN  [JS202011CQN]
TP1  TESTPOINT_BIG  [TP1]
TP2  TESTPOINT_BIG  [TP1]
TP7  TESTPOINT_BIG  [TP1]
TP8  TESTPOINT_BIG  [TP1]
TP9  TESTPOINT_BIG  [TP1]
TP10  TESTPOINT_BIG  [TP1]
TP13  TESTPOINT_BIG  [TP1]
TP14  TESTPOINT_BIG  [TP1]
TP15  TESTPOINT_BIG  [TP1]
TP16  TESTPOINT_BIG  [TP1]
U5  LTC3604IUD  [QFN16_3X3]
U7  LTC4415IMSE  [MSOP16_EXP]
U8  LTC4313CMS8  [MSOP-8]
U13  MCP23008-E/ML  [QFN20]
U14  24AA02T-I/OT  24AA64  [SOT-23-5]
U15  LT6654BMPS6-1.25  LTC6654SOT23-6  [SOT-23-6]

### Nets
+3V3: C20.1 R24.R1_2 R24.R2_2 R24.R3_2 R24.R4_2 R25.1 R35.1 R57.1 R58.1 R60.1 U8.8 U13.18 ; also sheet 3
+12V: C9.2 C32.+ J1.3 JP1.13 JP1.14 JP2.13 JP2.14 U5.14 U5.15 U5.16
A0_MUX: JP3.6 R24.R2_1 U13.3
A1_MUX: JP3.7 R24.R3_1 U13.2
A2_MUX: JP3.8 R24.R4_1 U13.1
ALERTB: JP1.3 JP2.3 TP10.TP ; also sheet 3
CH7_SHORT: R61.2 ; also sheet 3
CTRL: C26.1 JP1.2 JP2.2 R88.2 S1.2(B:P) S1.5(A:P) ; also sheet 3
CTRL_P: R88.1 TP8.TP
EESCL: J2.11 R30.1 U14.1
EESDA: J2.12 R36.1 U14.3
EEVCC: C15.1 C25.1 C41.1 D1.2 J2.1 JP1.8 JP2.8 R30.2 R36.2 U7.7 U7.8 U14.4
FAULTB: JP1.1 JP2.1 TP9.TP ; also sheet 3
FB_LTC3604: C11.2 C14.1 R14.2 R15.1 U5.11
GND: C9.1 C13.2 C14.2 C15.2 C16.2 C20.2 C25.2 C26.2 C27.2 C32.- C41.2 C42.2 C43.1 C45.2 C47.2 C48.2 C49.2 J1.1 J1.2 J2.3 J2.10 JP1.11 JP1.12 JP2.11 JP2.12 JP3.1 JP3.2 JP3.3 LED3.N(C) R14.1 R19.1 R20.1 R21.1 S1.3(B:S) S1.6(A:S) TP1.TP TP2.TP TP16.TP U5.9 U5.PAD U7.EXP U8.4 U13.17 U13.PAD U14.2 U14.5 U15.1 U15.2 ; also sheet 1,2,3
IBV_AUX: C11.1 C13.1 C16.1 D1.1 L5.2 R15.2 R17.2 U5.8 U7.1 U7.2
INTVCC_LTC3604: C47.1 U5.1 U5.7 U5.10
ITH_LTC3604: C48.1 R71.2 U5.12
N$1: C42.1 D1.3 U15.4
N$4: R61.1 U13.16
N$16: JP3.4 R57.2
N$61: C49.1 R71.1
N$63: LED3.P(A) R16.1
N$64: R21.2 R63.1 U7.5
N$66: C27.1 R25.2 U13.4
N$68: R20.2 U7.4
N$69: R17.1 R19.2 U7.3 U7.6
N$70: C10.2 U5.6
N$74: R35.2 U8.1 U13.9
RESETB: JP1.7 JP2.7 ; also sheet 3
SCL: TP13.TP U8.2 ; also sheet 3
SCL_IN: J2.4 JP1.6 JP2.6 R58.2 U8.3 U13.19
SDA: TP15.TP U8.7 ; also sheet 3
SDA_IN: J2.2 JP1.4 JP2.4 R60.2 U8.6 U13.20
SHARE_CLK: JP1.5 JP2.5 JP3.5 TP7.TP ; also sheet 3
SW_LTC3604: C10.1 L5.1 U5.3 U5.4
UNUSED1: JP1.9 JP2.9
UNUSED2: JP1.10 JP2.10
VDD: C45.1 R16.2 TP14.TP U7.9 U7.10 U7.15 U7.16 ; also sheet 1,2,3
VREF: C43.2 R63.2 U15.6
Unconnected: J2.5 J2.6 J2.7 J2.8 J2.9 R24.R1_1 S1.1(B:O) S1.4(A:O) U5.2 U5.5 U5.13 U7.11 U7.12 U7.13 U7.14 U8.5 U13.5 U13.6 U13.7 U13.8 U13.10 U13.11 U13.12 U13.13 U13.14 U13.15 U15.3 U15.5

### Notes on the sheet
- 1 | PRODUCTION | MIKE P. | 06-18-13
- RUN
- OFF
- 1206 | 6-14V
- 7343
- POWER INPUT
- IHLP-1616BZ
- 1210
- 1206
- 1210
- R. S.
- NOTES: UNLESS OTHERWISE SPECIFIED:
- MIKE P.
- 1. ALL RESISTORS ARE 1% 0603.
- LTC2977CUP 8-CHANNEL
- 2. ALL CAPACITORS ARE 16V 0603. | POWER SYSTEM MANAGER
- 3. THE INTERMEDIATE BUS IS VDD=5.0V | LTC2977
- DEMO CIRCUIT 2028A | 1

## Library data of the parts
C1-C31 C33-C57 = kalin:C: CAPACITOR, European symbol
C32 = kalin:CPOL: Polarized Capacitor
D1 = kalin:BAT30CWFILM: Small signal dual schottky diode (common cathode)
J1 = kalin:PJ-002A: Power Jack from CUI Inc. PJ-002A
J2 = kalin:CONN_DC1613: Connector for LT DC1613 USB Dongle
JP1 JP2 = pinhead_2mm:PINHD-2X07: PIN HEADER
JP3 = kalin:TDA04H0SK1: Ultra-miniature Surface Mount Half-pitch DIP Switch
L1-L9 = kalin:L: Inductor
LED1-LED3 P1-P8 = kalin:LED-0603: SMD LED in R0603
Q1-Q9 = kalin:SI1304: N-Channel 30 V (D-S) MOSFET
R1-R12 R14-R23 R25-R58 R60-R63 R67 R68 R71-R88 = kalin:R: RESISTOR, American symbol
R24 R59 = kalin:R_ARRAY_4X_CRA06S: Thick Film Resistor Array
S1 = kalin:JS202011CQN: SLIDING SWITCH Siemens, distributor Buerklin, 11G766
SW1 SW2 = kalin:SWITCH_PTS635: PTS635SL25 Surface Mount Tactile Switch
TP1-TP20 = kalin:TESTPOINT_BIG: Large Test Point
U1-U4 U9-U12 = kalin:LTC3405: 1.5MHz, 300mA Synchronous Step-Down Regulator in ThinSOT
U5 = kalin:LTC3604: 2.5A, 15V Monolithic Synchronous Step-Down Regulator
U6 = kalin:LTC2978: Octal Digital Power Supply Manager with EEPROM
U7 = kalin:LTC4415: Dual 4A Ideal Diodes with Adjustable Current Limit
U8 = kalin:LTC4313: 2-Wire Bus Buffers with High Noise Margin
U13 = kalin:MCP23008: I2C 8-pin IO Expander
U14 = kalin:24AA64: 64K I2C? Serial EEPROM
U15 = kalin:LTC6654: SOT-23 Precision Wide Supply High Output Drive Low Noise Reference
U16 = kalin:SN74LVC2G34: DUAL BUFFER GATE
VSNSN1-VSNSN24 = kalin:TESPOINT_SMD: SMALL SMD Test Point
